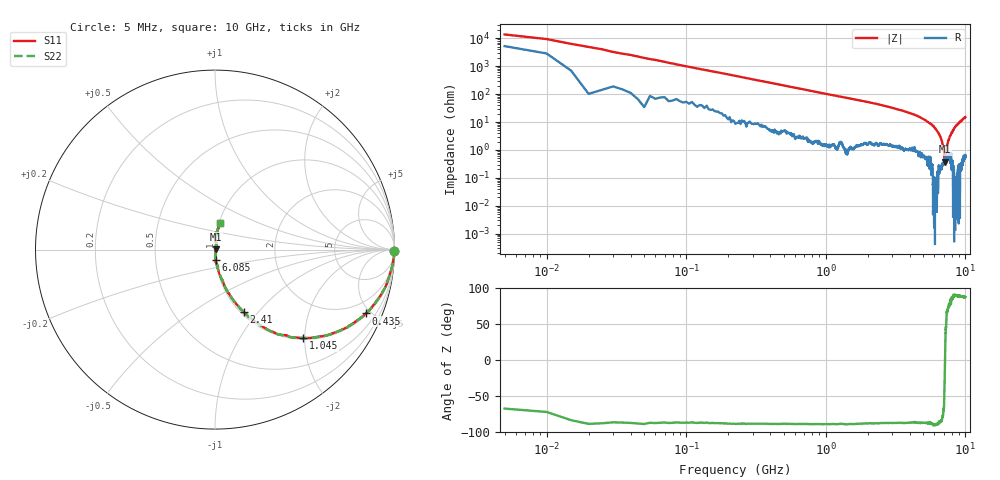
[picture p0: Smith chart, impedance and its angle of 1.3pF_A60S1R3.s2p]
! Amotech Co.,Ltd.
! http://www.amotech.co.kr/
! Part Number: A60S1R3
! These Parameters are Measured in Series Mode Connection
! Operation Temp=25[degC], DC Bias Voltage=0[V]
! Freq. Start=5[MHz] Stop=10[GHz], 2000[Steps]
! Date: Monday, July 13, 2020, 01:49:57
# GHZ S RI R 50.000000
!Freq.(Hz) S11(Real) S11(Imag) S21(Real) S21(Imag) S12(Real) S12(Imag) S22(Real) S22(Imag)
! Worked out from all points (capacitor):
!   2000 points, 5 MHz to 10 GHz, reference 50 ohm
!   read as one part in series: C = 1.61 pF near 55 MHz
!   lowest |Z| = 378 mohm at 7.18 GHz (marker M1)
!   series resonance near 7.146 GHz, so ESL is about 310 pH
!   S11 on the Smith chart (normalised r, x): 5 MHz: open; 435 MHz: 1.09, -4.70; 1.045 GHz: 1.03, -1.97; 2.41 GHz: 1.03, -0.84; 6.085 GHz: 1.00, -0.12; 10 GHz: 1.01, +0.30
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0.005  0.9972 -0.00675  0.00285 0.00675  0.00285 0.00675  0.9972 -0.00675
0.075  0.9911 -0.0751  0.00889 0.0751  0.00889 0.0751  0.9911 -0.0751
0.135  0.9764 -0.1319  0.0236 0.1319  0.0236 0.1319  0.9764 -0.1319
0.26  0.932 -0.238  0.068 0.238  0.068 0.238  0.932 -0.238
0.435  0.8417 -0.3554  0.1583 0.3554  0.1583 0.3554  0.8417 -0.3554
0.705  0.6754 -0.459  0.3246 0.459  0.3246 0.459  0.6754 -0.459
1.045  0.4916 -0.4936  0.5084 0.4936  0.5084 0.4936  0.4916 -0.4936
1.675  0.2815 -0.4386  0.7185 0.4386  0.7185 0.4386  0.2815 -0.4386
2.41  0.16 -0.3495  0.84 0.3495  0.84 0.3495  0.16 -0.3495
3.34  0.082 -0.2502  0.918 0.2502  0.918 0.2502  0.082 -0.2502
5.005  0.0217 -0.1235  0.9783 0.1235  0.9783 0.1235  0.0217 -0.1235
6.085  0.00283 -0.0594  0.9972 0.0594  0.9972 0.0594  0.00283 -0.0594
6.67  0.00315 -0.0262  0.9968 0.0262  0.9968 0.0262  0.00315 -0.0262
6.865  0.00347 -0.0158  0.9965 0.0158  0.9965 0.0158  0.00347 -0.0158
7.13  0.00449 -0.000524  0.9955 0.000524  0.9955 0.000524  0.00449 -0.000524
7.18  0.00348 0.00144  0.9965 -0.00144  0.9965 -0.00144  0.00348 0.00144
7.275  0.00588 0.00645  0.9941 -0.00645  0.9941 -0.00645  0.00588 0.00645
7.355  0.00517 0.0112  0.9948 -0.0112  0.9948 -0.0112  0.00517 0.0112
7.55  0.00672 0.0213  0.9933 -0.0213  0.9933 -0.0213  0.00672 0.0213
7.93  0.00582 0.0402  0.9942 -0.0402  0.9942 -0.0402  0.00582 0.0402
8.335  0.00261 0.061  0.9974 -0.061  0.9974 -0.061  0.00261 0.061
10  0.0279 0.1461  0.9721 -0.1461  0.9721 -0.1461  0.0279 0.1461
